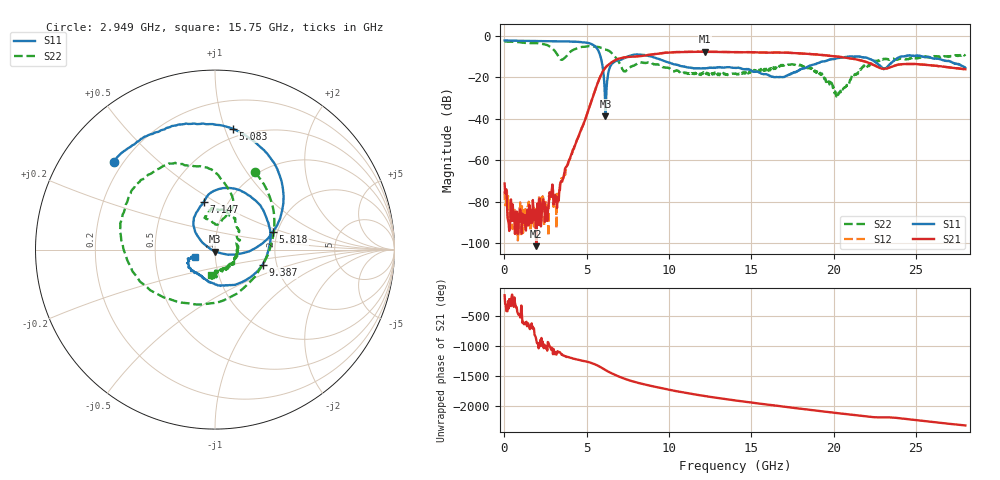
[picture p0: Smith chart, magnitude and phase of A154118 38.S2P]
!  2-Port S-parameters saved by WinCal
! VAR MeasName=S-Parameters (CALIBRATED_DATA) read from VNA (N5230A)
! VAR MeasDate=2015-9-10 14:37:21
! VAR NAME=A154118 38
! VAR FILENAME=A154118 38.S2P
! VAR DATE=2015-9-10 14:37:21
! VAR PHYS_PORTS=1,2
# Hz S DB R 50
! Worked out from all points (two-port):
!   801 points, 10 MHz to 28 GHz, reference 50 ohm
!   highest |S21| = -7.61 dB at 12.19 GHz (marker M1); lowest = -101.6 dB at 1.934 GHz (marker M2)
!   |S21| within 3 dB of the highest: 7.105 GHz to 20.83 GHz (13.73 GHz wide, 98.3 % of centre)
!   lowest |S11| = -38.7 dB at 6.133 GHz (marker M3), VSWR 1.02, Z = 50.2 - j1.14 ohm
!   |S11| at or under -10 dB: 8.957 GHz to 20.83 GHz (11.87 GHz wide, 79.7 % of centre); 21.58 GHz to 24.04 GHz (2.456 GHz wide, 10.8 % of centre); 25.46 GHz to end of sweep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
!   |S22| runs from -29.2 to -2.7 dB; largest |S21 - S12| = 0.0084
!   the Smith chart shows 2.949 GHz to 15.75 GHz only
!   S11 on the Smith chart (normalised r, x): 2.949 GHz: 0.16, +0.36; 5.083 GHz: 0.43, +1.07; 5.818 GHz: 1.89, +0.42; 7.147 GHz: 0.77, +0.45; 9.387 GHz: 1.69, -0.31; 15.75 GHz: 0.80, -0.06
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1e7  -2.16 179.7  -71.31 -151.8  -75.09 159.1  -2.67 179.8
2.899e8  -2.19 175.7  -94.22 144.0  -87.71 70.7  -2.71 172.9
1.934312e9  -2.42 154.6  -101.57 -176.8  -83.86 150.4  -3.44 130.6
2.94895e9  -2.54 139.2  -74.56 -54.0  -77.22 -61.2  -6.29 62.4
3.158875e9  -2.50 135.5  -80.15 -60.6  -92.89 -63.6  -8.26 31.9
3.683688e9  -2.62 125.1  -63.95 -86.3  -67.19 -82.4  -10.42 -95.6
4.698325e9  -3.02 98.2  -44.43 -160.4  -44.38 -160.7  -5.29 165.8
5.083188e9  -3.34 81.5  -36.03 177.0  -36.00 177.4  -4.97 146.5
5.817925e9  -9.44 17.0  -19.72 93.9  -19.67 94.1  -5.48 114.6
6.132812e9  -38.74 -80.1  -15.31 42.5  -15.25 42.4  -6.52 100.2
6.482688e9  -13.92 126.1  -12.93 -8.0  -12.87 -8.2  -7.97 85.8
7.14745e9  -11.22 102.8  -10.53 -87.2  -10.50 -87.5  -15.80 77.7
8.162088e9  -8.95 60.7  -9.73 -173.8  -9.68 -173.9  -13.08 96.6
9.351662e9  -11.06 -15.3  -8.58 111.3  -8.49 111.2  -13.79 58.1
9.38665e9  -11.11 -17.8  -8.50 109.5  -8.45 109.3  -13.91 56.5
1.218565e10  -15.59 -128.3  -7.61 -31.1  -7.57 -31.7  -17.45 -38.8
1.4005e10  -15.38 -151.6  -7.84 -102.9  -7.80 -103.4  -18.31 -85.7
1.575438e10  -18.51 -160.2  -8.00 -165.2  -7.96 -165.7  -16.80 -98.1
1.869332e10  -13.91 -118.0  -8.77 95.1  -8.76 94.7  -15.82 -143.2
2.019779e10  -10.73 -133.5  -9.98 46.1  -9.89 45.2  -27.71 -130.7
2.334666e10  -14.26 -136.4  -15.35 -25.0  -15.35 -26.0  -11.40 -94.3
2.8e10  -15.38 172.7  -16.06 -160.2  -16.14 -161.0  -8.89 -119.2
